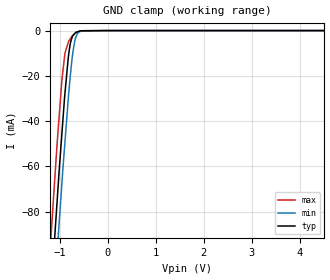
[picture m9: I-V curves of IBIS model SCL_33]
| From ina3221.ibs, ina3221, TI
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|   SCL input model
[Model]   SCL_33
Model_type   Input
Vinl = 0.99   |min, GND -0.5 V
Vinh = 2.31   |max. V+ 6 V
|   typ   min   max
|   (nom PVT)   (Fast PVT)   (slow PVT)
C_comp   1.432E-12   1.406E-12   1.452E-12
| Where   nom PVT is  Nominal Process, 3.3V, 25C
|   Fast PVT is Strong Process, 3.6V, -40C
|   Slow PVT is Weak Process, 3.0V, 85C
|C_comp - from L-C Tank method, L = 1nH, peak frequency
[Model Spec]
| variable   typ   min   max
Vinl   0.99   0.9   1.08
Vinh   2.31   2.1   2.52
|Vinl = 0.3 x V+, Vinh = 0.7 x V+
[Voltage Range]   3.3   3   3.6
|Ambient Temperature Range   27   85   -40
[Temperature Range]   30   88   -40
[Power Clamp Reference]   3.3   3   3.6
[GND Clamp Reference]   0   0   0
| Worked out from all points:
|   GND clamp passes 1 mA (typ) near -0.68 V on its own axis
[GND Clamp]
|   Voltage   I(typ)   I(min)   I(max)
-3.3V     -844mA     -857.5mA   -829.4mA
-1.178V   -113.6mA   -136.5mA   -88.56mA
-1.081V   -82.98mA   -105.4mA   -57.55mA
-1.058V   -75.46mA   -98.06mA   -49.93mA
-1.016V   -62.15mA   -85.21mA   -38.11mA
-956.3mV  -45.06mA   -67.06mA   -21.53mA
-894.2mV  -27.66mA   -49.23mA   -9.937mA
-783.7mV  -5.949mA   -20.19mA   -3.618mA
-727.7mV  -2.225mA   -9.444mA   -2.096mA
-669.5mV  -802.1uA   -3.102mA   -987.5uA
-49.19mV  -3.606uA   0A         -543.5nA
6.59V     0A         0A         0A
[POWER Clamp]
|   SCR cell for ESD function. Effects occurr above VDD x 2
|   Voltage   I(typ)   I(min)   I(max)
-3.3V     0A         0A         0A
0V        0A         0A         0A
6.6V      0A         0A         0A
